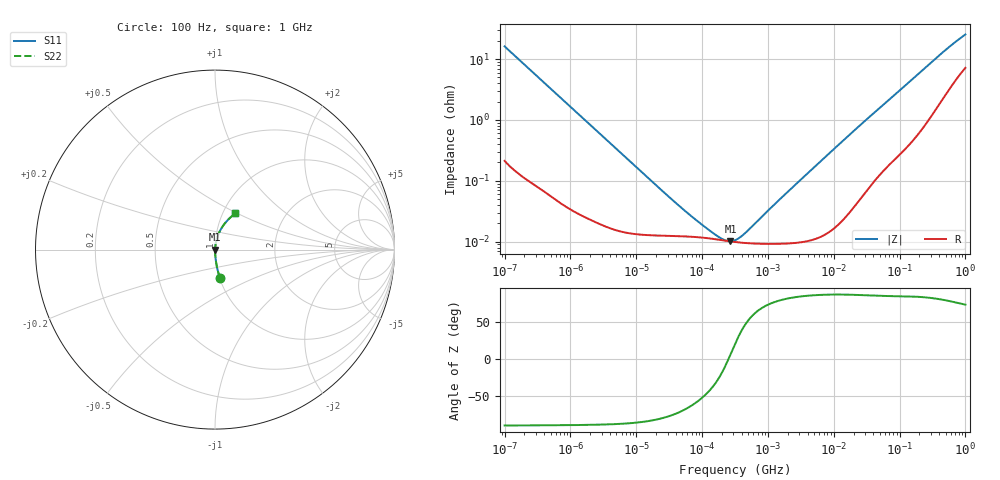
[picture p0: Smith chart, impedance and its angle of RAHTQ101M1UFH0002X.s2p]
! RAHTQ101M1UFH0002X  S-PARAMETER MODEL  (AEC-Q200 qualified)
! Model Generated by ELNA Corporation (http://www.ty-top.com)
! Version 1.0
! ELNA Control No. 231222
! Copyright (c) 2023 ELNA CO.,LTD. All Rights Reserved.
! Products Name : CONDUCTIVE POLYMER HYBRID ALUMINUM ELECTROLYTIC CAPACITORS
! Characteristics :
!  Capacitance  :  100uF  ,  Rated voltage  :  50V
!  Operating Temp. Range  :  -55 to +150 degC  ,  Endurance  :  1000hr at 150 degC
!  Dimension D  :  10mm  ,  Dimension L  :  10mm
! Frequency Range : 100Hz - 1GHz
! External Node Assignments :
!  1  o---| |---o  2
# MHz S RI R 50
!Freq[MHz].  S11 Real  S11 Imag  S21 Real  S21 Imag  S12 Real  S12 Imag  S22 Real  S22 Imag
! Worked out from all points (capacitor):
!   401 points, 100 Hz to 1 GHz, reference 50 ohm
!   read as one part in series: C = 98.1 uF near 108 Hz
!   lowest |Z| = 10.1 mohm at 269.2 kHz (marker M1)
!   series resonance near 251.1 kHz, so ESL is about 4.1 nH
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0.0001  0.0276 -0.1573  0.9724 0.1573  0.9724 0.1573  0.0276 -0.1573
0.000113  0.022 -0.1403  0.978 0.1403  0.978 0.1403  0.022 -0.1403
0.000183  0.00897 -0.0879  0.991 0.0879  0.991 0.0879  0.00897 -0.0879
0.000309  0.00357 -0.0525  0.9964 0.0525  0.9964 0.0525  0.00357 -0.0525
0.001488  0.000391 -0.0111  0.9996 0.0111  0.9996 0.0111  0.000391 -0.0111
0.022131  0.000126 -0.000754  0.9999 0.000754  0.9999 0.000754  0.000126 -0.000754
0.05821  0.000122 -0.000279  0.9999 0.000279  0.9999 0.000279  0.000122 -0.000279
0.130317  0.000113 -0.000102  0.9999 0.000102  0.9999 0.000102  0.000113 -0.000102
0.203002  0.000105 -3.25e-05  0.9999 3.25e-05  0.9999 3.25e-05  0.000105 -3.25e-05
0.238506  0.000103 -7.92e-06  0.9999 7.92e-06  0.9999 7.92e-06  0.000103 -7.92e-06
0.269153  0.000101 1.09e-05  0.9999 -1.09e-05  0.9999 -1.09e-05  0.000101 1.09e-05
0.316228  9.86e-05 3.68e-05  0.9999 -3.68e-05  0.9999 -3.68e-05  9.86e-05 3.68e-05
0.371535  9.67e-05 6.43e-05  0.9999 -6.43e-05  0.9999 -6.43e-05  9.67e-05 6.43e-05
0.454465  9.48e-05 0.000102  0.9999 -0.000102  0.9999 -0.000102  9.48e-05 0.000102
1.348963  9.2e-05 0.00043  0.9999 -0.00043  0.9999 -0.00043  9.2e-05 0.00043
4.704354  0.000109 0.00155  0.9999 -0.00155  0.9999 -0.00155  0.000109 0.00155
21.75204  0.000456 0.0071  0.9995 -0.0071  0.9995 -0.0071  0.000456 0.0071
69.9842  0.0023 0.0216  0.9977 -0.0216  0.9977 -0.0216  0.0023 0.0216
184.0772  0.0084 0.0538  0.9916 -0.0538  0.9916 -0.0538  0.0084 0.0538
429.0422  0.0335 0.1151  0.9665 -0.1151  0.9665 -0.1151  0.0335 0.1151
695.825  0.0708 0.1644  0.9292 -0.1644  0.9292 -0.1644  0.0708 0.1644
1000  0.1131 0.2019  0.8869 -0.2019  0.8869 -0.2019  0.1131 0.2019
